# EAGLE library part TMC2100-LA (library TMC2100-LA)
Universal high voltage driver for two-phase bipolar stepper motor, Step/Dir, QFN36_5x6
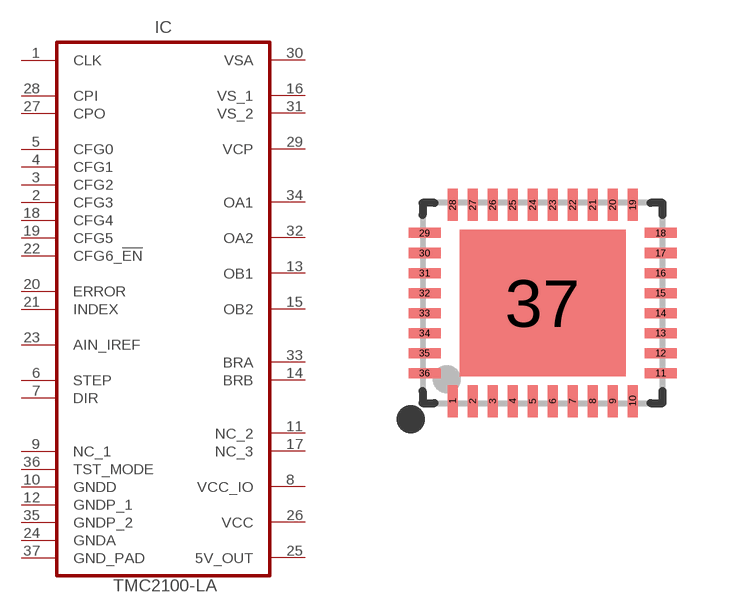
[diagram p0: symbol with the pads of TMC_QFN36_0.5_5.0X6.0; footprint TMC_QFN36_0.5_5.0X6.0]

Designator prefix IC

## TMC2100-LA (DATASHEET: http://www_trinamic_com/_scripts/download_php?file=_articles%2Fproducts%2Fintegrated-circuits%2Ftmc2100%2F_datasheet%2FTMC2100_datasheet_pdf; DESCRIPTION: Universal high voltage driver for two-phase bipolar stepper motor, Step/Dir, QFN36_5x6; DISTRIBUTOR1: Digikey; GEOMETRY_HEIGHT: 0_9mm; MANUFACTURER: TRINAMIC; ORDERCODE-DISTRI1: 1460-1128-1-ND; ORDERCODE-MANU1: TMC2100-LA; VALUE: TMC2100-LA)  [TMC_QFN36_0.5_5.0X6.0]
1  CLK  in
2  CFG3  in
3  CFG2  in
4  CFG1  in
5  CFG0  in
6  STEP  in
7  DIR  in
8  VCC_IO  pwr
9  NC_1  pas
10  GNDD  pwr
11  NC_2  pas
12  GNDP_1  pwr
13  OB1  out
14  BRB  out
15  OB2  out
16  VS_1  pwr
17  NC_3  pas
18  CFG4  in
19  CFG5  in
20  ERROR  oc
21  INDEX  oc
22  CFG6_!EN  in
23  AIN_IREF  in
24  GNDA  pwr
25  5V_OUT  pwr
26  VCC  pwr
27  CPO  in
28  CPI  in
29  VCP  pwr
30  VSA  pwr
31  VS_2  pwr
32  OA2  out
33  BRA  out
34  OA1  out
35  GNDP_2  pwr
36  TST_MODE  in
37  GND_PAD  pwr

## Footprint TMC_QFN36_0.5_5.0X6.0 (pad centres in mm)
smd 0.25 x 0.8: 1 -2.25,-2.45; 2 -1.75,-2.45; 3 -1.25,-2.45; 4 -0.75,-2.45; 5 -0.25,-2.45; 6 0.25,-2.45; 7 0.75,-2.45; 8 1.25,-2.45; 9 1.75,-2.45; 10 2.25,-2.45; 19 2.25,2.45; 20 1.75,2.45; 21 1.25,2.45; 22 0.75,2.45; 23 0.25,2.45; 24 -0.25,2.45; 25 -0.75,2.45; 26 -1.25,2.45; 27 -1.75,2.45; 28 -2.25,2.45
smd 0.8 x 0.25: 11 2.95,-1.75; 12 2.95,-1.25; 13 2.95,-0.75; 14 2.95,-0.25; 15 2.95,0.25; 16 2.95,0.75; 17 2.95,1.25; 18 2.95,1.75; 29 -2.95,1.75; 30 -2.95,1.25; 31 -2.95,0.75; 32 -2.95,0.25; 33 -2.95,-0.25; 34 -2.95,-0.75; 35 -2.95,-1.25; 36 -2.95,-1.75
smd 4.15 x 3.65: 37 0,0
